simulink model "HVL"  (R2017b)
settings: Solver=FixedStepDiscrete  StartTime=0.0  StopTime=10.0  FixedStep=0.01  RelTol=1e-3  EnableMultiTasking=on
undefined symbols (not defined in the file): ASWTYPE_FALSE, ASWTYPE_TRUE, CcHVL_HvilSTGDutyThrd_pct, CcHVL_HvilSTVDutyThrd_pct, CcHVL_HVLSelfCheckTime_ms, CcHVL_PWMHighDuty_pct, CcHVL_PWMInHighPer_ms, CcHVL_PWMInLowPer_ms, CcHVL_PWMLowDuty_pct, CcHVL_PWMOutDuty_pct, CcHVL_PWMOutPer_us, Enum_MSMBMUState, HVL_CONST0_NUMB, HVL_CONST8_NUMB, HVL_CONST9_NUMB, HVL_RUNTIME_MS
libraries: AIWAYS_Powertrain_BMS_lib x11, simulink x1

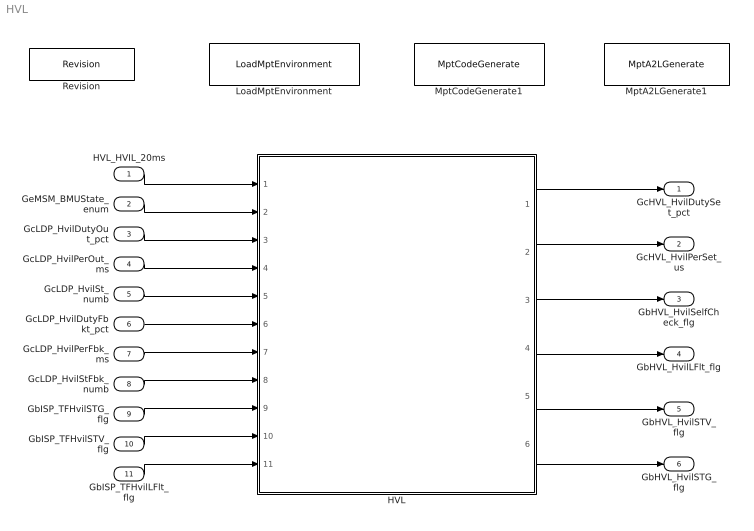
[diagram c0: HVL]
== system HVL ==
  HVL_HVIL_20ms : Inport
  GeMSM_BMUState_enum : Inport  Port=2
  GcLDP_HvilDutyOut_pct : Inport  Port=3
  GcLDP_HvilPerOut_ms : Inport  Port=4
  GcLDP_HvilSt_numb : Inport  Port=5
  GcLDP_HvilDutyFbkt_pct : Inport  Port=6
  GcLDP_HvilPerFbk_ms : Inport  Port=7
  GcLDP_HvilStFbk_numb : Inport  Port=8
  GbISP_TFHvilSTG_flg : Inport  Port=9
  GbISP_TFHvilSTV_flg : Inport  Port=10
  GbISP_TFHvilLFlt_flg : Inport  Port=11
  HVL : Subsystem
  LoadMptEnvironment : AIWAYS_Powertrain_BMS_lib/Config/LoadMptEnvironment  ProjectName=Comm  SuppierID=NewPlatformUAES
  MptA2LGenerate1 : AIWAYS_Powertrain_BMS_lib/Config/MptA2LGenerate  SystemSampleTime=-1
  MptCodeGenerate1 : AIWAYS_Powertrain_BMS_lib/Config/MptCodeGenerate  SystemSampleTime=-1
  Revision : AIWAYS_Powertrain_BMS_lib/Config/Revision  curVersion='M100C100'  newVersion='M100C100'
  GcHVL_HvilDutySet_pct : Outport
  GcHVL_HvilPerSet_us : Outport  Port=2
  GbHVL_HvilSelfCheck_flg : Outport  Port=3
  GbHVL_HvilLFlt_flg : Outport  Port=4
  GbHVL_HvilSTV_flg : Outport  Port=5
  GbHVL_HvilSTG_flg : Outport  Port=6
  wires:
  HVL_HVIL_20ms/1 -> HVL/1(HVL_HVIL_20ms)
  GeMSM_BMUState_enum/1 -> HVL/2(GeMSM_BMUState_enum)
  GcLDP_HvilDutyOut_pct/1 -> HVL/3(GcLDP_HvilDutyOut_pct)
  GcLDP_HvilPerOut_ms/1 -> HVL/4(GcLDP_HvilPerOut_ms)
  GcLDP_HvilSt_numb/1 -> HVL/5(GcLDP_HvilSt_numb)
  GcLDP_HvilDutyFbkt_pct/1 -> HVL/6(GcLDP_HvilDutyFbkt_pct)
  GcLDP_HvilPerFbk_ms/1 -> HVL/7(GcLDP_HvilPerFbk_ms)
  GcLDP_HvilStFbk_numb/1 -> HVL/8(GcLDP_HvilStFbk_numb)
  HVL/1(GcHVL_HvilDutySet_pct) -> GcHVL_HvilDutySet_pct/1
  HVL/2(GcHVL_HvilPerSet_us) -> GcHVL_HvilPerSet_us/1
  HVL/3(GbHVL_HvilSelfCheck_flg) -> GbHVL_HvilSelfCheck_flg/1
  HVL/4(GbHVL_HvilLFlt_flg) -> GbHVL_HvilLFlt_flg/1
  HVL/5(GbHVL_HvilSTV_flg) -> GbHVL_HvilSTV_flg/1
  HVL/6(GbHVL_HvilSTG_flg) -> GbHVL_HvilSTG_flg/1
  GbISP_TFHvilSTG_flg/1 -> HVL/9(GbISP_TFHvilSTG_flg)
  GbISP_TFHvilSTV_flg/1 -> HVL/10(GbISP_TFHvilSTV_flg)
  GbISP_TFHvilLFlt_flg/1 -> HVL/11(GbISP_TFHvilLFlt_flg)

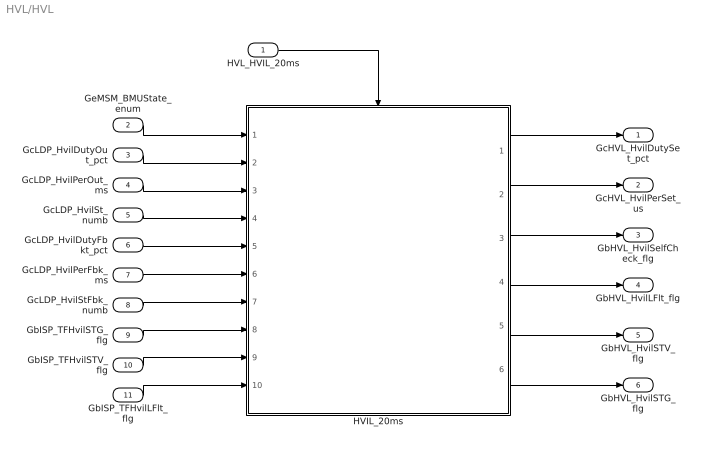
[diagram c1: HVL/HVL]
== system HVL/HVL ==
  HVL_HVIL_20ms : Inport
  GeMSM_BMUState_enum : Inport  Port=2
  GcLDP_HvilDutyOut_pct : Inport  Port=3
  GcLDP_HvilPerOut_ms : Inport  Port=4
  GcLDP_HvilSt_numb : Inport  Port=5
  GcLDP_HvilDutyFbkt_pct : Inport  Port=6
  GcLDP_HvilPerFbk_ms : Inport  Port=7
  GcLDP_HvilStFbk_numb : Inport  Port=8
  GbISP_TFHvilSTG_flg : Inport  Port=9
  GbISP_TFHvilSTV_flg : Inport  Port=10
  GbISP_TFHvilLFlt_flg : Inport  Port=11
  HVIL_20ms : Subsystem
  GcHVL_HvilDutySet_pct : Outport
  GcHVL_HvilPerSet_us : Outport  Port=2
  GbHVL_HvilSelfCheck_flg : Outport  Port=3
  GbHVL_HvilLFlt_flg : Outport  Port=4
  GbHVL_HvilSTV_flg : Outport  Port=5
  GbHVL_HvilSTG_flg : Outport  Port=6
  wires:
  HVL_HVIL_20ms/1 -> HVIL_20ms/Trigger
  GeMSM_BMUState_enum/1 -> HVIL_20ms/1(GeMSM_BMUState_enum)
  GcLDP_HvilDutyOut_pct/1 -> HVIL_20ms/2(GcLDP_HvilDutyOut_pct)
  GcLDP_HvilPerOut_ms/1 -> HVIL_20ms/3(GcLDP_HvilPerOut_ms)
  GcLDP_HvilSt_numb/1 -> HVIL_20ms/4(GcLDP_HvilSt_numb)
  GcLDP_HvilDutyFbkt_pct/1 -> HVIL_20ms/5(GcLDP_HvilDutyFbkt_pct)
  GcLDP_HvilPerFbk_ms/1 -> HVIL_20ms/6(GcLDP_HvilPerFbk_ms)
  GcLDP_HvilStFbk_numb/1 -> HVIL_20ms/7(GcLDP_HvilStFbk_numb)
  HVIL_20ms/3(GbHVL_HvilSelfCheck_flg) -> GbHVL_HvilSelfCheck_flg/1
  HVIL_20ms/2(GcHVL_HvilPerSet_us) -> GcHVL_HvilPerSet_us/1
  HVIL_20ms/4(GbHVL_HvilLFlt_flg) -> GbHVL_HvilLFlt_flg/1
  HVIL_20ms/1(GcHVL_HvilDutySet_pct) -> GcHVL_HvilDutySet_pct/1
  HVIL_20ms/5(GbHVL_HvilSTV_flg) -> GbHVL_HvilSTV_flg/1
  HVIL_20ms/6(GbHVL_HvilSTG_flg) -> GbHVL_HvilSTG_flg/1
  GbISP_TFHvilSTG_flg/1 -> HVIL_20ms/8(GbISP_TFHvilSTG_flg)
  GbISP_TFHvilSTV_flg/1 -> HVIL_20ms/9(GbISP_TFHvilSTV_flg)
  GbISP_TFHvilLFlt_flg/1 -> HVIL_20ms/10(GbISP_TFHvilLFlt_flg)

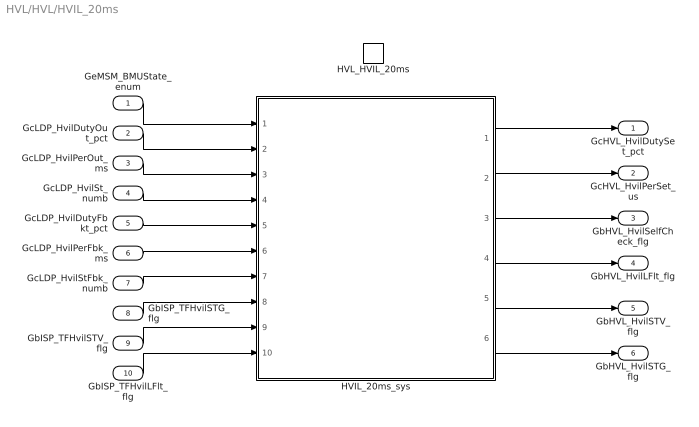
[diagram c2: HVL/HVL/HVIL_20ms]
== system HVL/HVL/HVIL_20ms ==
  GeMSM_BMUState_enum : Inport
  GcLDP_HvilDutyOut_pct : Inport  Port=2
  GcLDP_HvilPerOut_ms : Inport  Port=3
  GcLDP_HvilSt_numb : Inport  Port=4
  GcLDP_HvilDutyFbkt_pct : Inport  Port=5
  GcLDP_HvilPerFbk_ms : Inport  Port=6
  GcLDP_HvilStFbk_numb : Inport  Port=7
  GbISP_TFHvilSTG_flg : Inport  Port=8
  GbISP_TFHvilSTV_flg : Inport  Port=9
  GbISP_TFHvilLFlt_flg : Inport  Port=10
  HVL_HVIL_20ms : TriggerPort  TriggerType=function-call  VariantControl=(inherit)
  HVIL_20ms_sys : Subsystem
  GcHVL_HvilDutySet_pct : Outport
  GcHVL_HvilPerSet_us : Outport  Port=2
  GbHVL_HvilSelfCheck_flg : Outport  Port=3
  GbHVL_HvilLFlt_flg : Outport  Port=4
  GbHVL_HvilSTV_flg : Outport  Port=5
  GbHVL_HvilSTG_flg : Outport  Port=6
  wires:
  GeMSM_BMUState_enum/1 -> HVIL_20ms_sys/1(GeMSM_BMUState_enum)
  GcLDP_HvilDutyOut_pct/1 -> HVIL_20ms_sys/2(GcLDP_HvilDutyOut_pct)
  GcLDP_HvilPerOut_ms/1 -> HVIL_20ms_sys/3(GcLDP_HvilPerOut_ms)
  GcLDP_HvilSt_numb/1 -> HVIL_20ms_sys/4(GcLDP_HvilSt_numb)
  GcLDP_HvilDutyFbkt_pct/1 -> HVIL_20ms_sys/5(GcLDP_HvilDutyFbkt_pct)
  GcLDP_HvilPerFbk_ms/1 -> HVIL_20ms_sys/6(GcLDP_HvilPerFbk_ms)
  GcLDP_HvilStFbk_numb/1 -> HVIL_20ms_sys/7(GcLDP_HvilStFbk_numb)
  HVIL_20ms_sys/1(GcHVL_HvilDutySet_pct) -> GcHVL_HvilDutySet_pct/1
  HVIL_20ms_sys/2(GcHVL_HvilPerSet_us) -> GcHVL_HvilPerSet_us/1
  HVIL_20ms_sys/3(GbHVL_HvilSelfCheck_flg) -> GbHVL_HvilSelfCheck_flg/1
  HVIL_20ms_sys/4(GbHVL_HvilLFlt_flg) -> GbHVL_HvilLFlt_flg/1
  HVIL_20ms_sys/5(GbHVL_HvilSTV_flg) -> GbHVL_HvilSTV_flg/1
  HVIL_20ms_sys/6(GbHVL_HvilSTG_flg) -> GbHVL_HvilSTG_flg/1
  GbISP_TFHvilSTG_flg/1 -> HVIL_20ms_sys/8(GbISP_TFHvilSTG_flg)
  GbISP_TFHvilSTV_flg/1 -> HVIL_20ms_sys/9(GbISP_TFHvilSTV_flg)
  GbISP_TFHvilLFlt_flg/1 -> HVIL_20ms_sys/10(GbISP_TFHvilLFlt_flg)

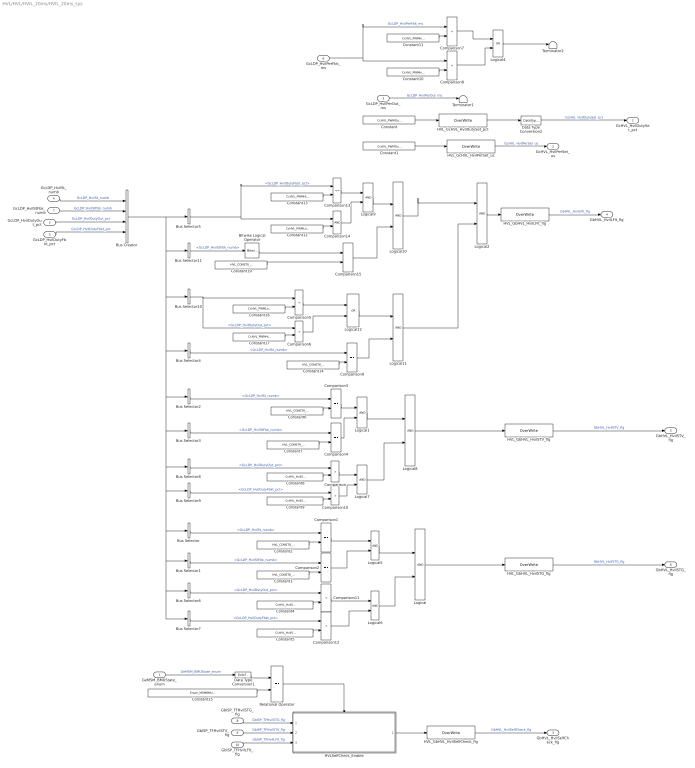
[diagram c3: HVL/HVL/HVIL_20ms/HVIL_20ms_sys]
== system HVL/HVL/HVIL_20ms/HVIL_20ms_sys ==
  GeMSM_BMUState_enum : Inport
  GcLDP_HvilDutyOut_pct : Inport  Port=2
  GcLDP_HvilPerOut_ms : Inport  Port=3
  GcLDP_HvilSt_numb : Inport  Port=4
  GcLDP_HvilDutyFbkt_pct : Inport  Port=5
  GcLDP_HvilPerFbk_ms : Inport  Port=6
  GcLDP_HvilStFbk_numb : Inport  Port=7
  GbISP_TFHvilSTG_flg : Inport  Port=8
  GbISP_TFHvilSTV_flg : Inport  Port=9
  GbISP_TFHvilLFlt_flg : Inport  Port=10
  Bitwise Logical Operator : simulink/Logic and Bit Operations/Bitwise Operator  logicop=AND  UseBitMask=on  BitMask=HVL_CONST24_NUMB  BitMaskRealWorld=Stored Integer
  Bus Creator : BusCreator  Inputs=4
  Bus Selector : BusSelector  OutputSignals=GcLDP_HvilSt_numb
  Bus Selector1 : BusSelector  OutputSignals=GcLDP_HvilStFbk_numb
  Bus Selector10 : BusSelector  OutputSignals=GcLDP_HvilDutyOut_pct
  Bus Selector11 : BusSelector  OutputSignals=GcLDP_HvilStFbk_numb
  Bus Selector2 : BusSelector  OutputSignals=GcLDP_HvilSt_numb
  Bus Selector3 : BusSelector  OutputSignals=GcLDP_HvilStFbk_numb
  Bus Selector4 : BusSelector  OutputSignals=GcLDP_HvilSt_numb
  Bus Selector5 : BusSelector  OutputSignals=GcLDP_HvilDutyFbkt_pct
  Bus Selector6 : BusSelector  OutputSignals=GcLDP_HvilDutyOut_pct
  Bus Selector7 : BusSelector  OutputSignals=GcLDP_HvilDutyFbkt_pct
  Bus Selector8 : BusSelector  OutputSignals=GcLDP_HvilDutyOut_pct
  Bus Selector9 : BusSelector  OutputSignals=GcLDP_HvilDutyFbkt_pct
  Comparison{,6,8,10} (4 alike) : RelationalOperator  Operator=>  OutDataTypeStr=boolean
  Comparison{1..4,9,15} (6 alike) : RelationalOperator  Operator===  OutDataTypeStr=boolean
  Comparison{5,7,11..12} (4 alike) : RelationalOperator  Operator=<  OutDataTypeStr=boolean
  Comparison13 : RelationalOperator  Operator=<=  OutDataTypeStr=boolean
  Comparison14 : RelationalOperator  OutDataTypeStr=boolean
  Constant : Constant  Value=CcHVL_PWMOutDuty_pct
  Constant1 : Constant  Value=CcHVL_PWMOutPer_us
  Constant10 : Constant  Value=CcHVL_PWMInHighPer_ms
  Constant11 : Constant  Value=CcHVL_PWMInLowPer_ms
  Constant12 : Constant  Value=CcHVL_PWMLowDuty_pct
  Constant13 : Constant  Value=CcHVL_PWMHighDuty_pct
  Constant14 : Constant  Value=HVL_CONST8_NUMB
  Constant15 : Constant  Value=Enum_MSMBMUState.Enum_MSMBMUState_Standby
  Constant16 : Constant  Value=CcHVL_PWMLowDuty_pct
  Constant17 : Constant  Value=CcHVL_PWMHighDuty_pct
  Constant19 : Constant  Value=HVL_CONST0_NUMB
  Constant2 : Constant  Value=HVL_CONST8_NUMB
  Constant3 : Constant  Value=HVL_CONST8_NUMB
  Constant4 : Constant  Value=CcHVL_HvilSTGDutyThrd_pct
  Constant5 : Constant  Value=CcHVL_HvilSTGDutyThrd_pct
  Constant6 : Constant  Value=HVL_CONST9_NUMB
  Constant7 : Constant  Value=HVL_CONST9_NUMB
  Constant8 : Constant  Value=CcHVL_HvilSTVDutyThrd_pct
  Constant9 : Constant  Value=CcHVL_HvilSTVDutyThrd_pct
  Data Type Conversion1 : DataTypeConversion
  Data Type Conversion2 : DataTypeConversion
  HVLSelfCheck_Enable : Subsystem
  HVL_GbHVL_HvilLFlt_flg : AIWAYS_Powertrain_BMS_lib/Signals/OverWrite  OverWrite_Value=CbHVL_HvilLFltOvr_flg  OverWrite_flag=CbHVL_HvilLFltOvrSwt_flg
  HVL_GbHVL_HvilSTG_flg : AIWAYS_Powertrain_BMS_lib/Signals/OverWrite  OverWrite_Value=CbHVL_HvilSTGOvr_flg  OverWrite_flag=CbHVL_HvilSTGOvrSwt_flg
  HVL_GbHVL_HvilSTV_flg : AIWAYS_Powertrain_BMS_lib/Signals/OverWrite  OverWrite_Value=CbHVL_HvilSTVOvr_flg  OverWrite_flag=CbHVL_HvilSTVOvrSwt_flg
  HVL_GbHVL_HvilSelfCheck_flg : AIWAYS_Powertrain_BMS_lib/Signals/OverWrite  OverWrite_Value=CbHVL_HvilSelfCheckOvr_flg  OverWrite_flag=CbHVL_HvilSelfCheckOvrSwt_flg
  HVL_GcHVL_HvilDutySet_pct : AIWAYS_Powertrain_BMS_lib/Signals/OverWrite  OverWrite_Value=CcHVL_HvilDutySetOvr_pct  OverWrite_flag=CbHVL_HvilDutySetOvrSwt_flg
  HVL_GcHVL_HvilPerSet_us : AIWAYS_Powertrain_BMS_lib/Signals/OverWrite  OverWrite_Value=CcHVL_HvilPerSetOvr_us  OverWrite_flag=CbHVL_HvilPerSetOvrSwt_flg
  Logical{,1..2,5..11} (10 alike) : Logic  OutDataTypeStr=boolean
  Logical12 : Logic  Operator=OR  OutDataTypeStr=boolean
  Logical4 : Logic  Operator=OR  OutDataTypeStr=boolean
  Relational Operator : RelationalOperator  Operator===  OutDataTypeStr=boolean
  Terminator1 : Terminator
  Terminator2 : Terminator
  GcHVL_HvilDutySet_pct : Outport
  GcHVL_HvilPerSet_us : Outport  Port=2
  GbHVL_HvilSelfCheck_flg : Outport  Port=3
  GbHVL_HvilLFlt_flg : Outport  Port=4
  GbHVL_HvilSTV_flg : Outport  Port=5
  GbHVL_HvilSTG_flg : Outport  Port=6
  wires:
  GeMSM_BMUState_enum/1 -> Data Type Conversion1/1  "GeMSM_BMUState_enum"
  GcLDP_HvilPerOut_ms/1 -> Terminator1/1  "GcLDP_HvilPerOut_ms"
  GcLDP_HvilSt_numb/1 -> Bus Creator/1  "GcLDP_HvilSt_numb"
  GcLDP_HvilDutyFbkt_pct/1 -> Bus Creator/4  "GcLDP_HvilDutyFbkt_pct"
  GcLDP_HvilPerFbk_ms/1 -> Comparison7/1, Comparison8/1  "GcLDP_HvilPerFbk_ms"
  GcLDP_HvilStFbk_numb/1 -> Bus Creator/2  "GcLDP_HvilStFbk_numb"
  Data Type Conversion2/1 -> GcHVL_HvilDutySet_pct/1  "GcHVL_HvilDutySet_pct"
  HVL_GcHVL_HvilPerSet_us/1 -> GcHVL_HvilPerSet_us/1  "GcHVL_HvilPerSet_us"
  HVL_GbHVL_HvilSelfCheck_flg/1 -> GbHVL_HvilSelfCheck_flg/1  "GbHVL_HvilSelfCheck_flg"
  HVL_GbHVL_HvilLFlt_flg/1 -> GbHVL_HvilLFlt_flg/1  "GbHVL_HvilLFlt_flg"
  HVL_GbHVL_HvilSTV_flg/1 -> GbHVL_HvilSTV_flg/1  "GbHVL_HvilSTV_flg"
  HVL_GbHVL_HvilSTG_flg/1 -> GbHVL_HvilSTG_flg/1  "GbHVL_HvilSTG_flg"
  Constant1/1 -> HVL_GcHVL_HvilPerSet_us/1
  HVLSelfCheck_Enable/1(GbHVL_HvilSelfCheck_flg) -> HVL_GbHVL_HvilSelfCheck_flg/1
  Logical2/1 -> HVL_GbHVL_HvilLFlt_flg/1
  Logical8/1 -> HVL_GbHVL_HvilSTV_flg/1
  Logical/1 -> HVL_GbHVL_HvilSTG_flg/1
  Constant2/1 -> Comparison1/2
  Constant3/1 -> Comparison2/2
  Comparison1/1 -> Logical5/1
  Comparison2/1 -> Logical5/2
  Bus Selector/1 -> Comparison1/1  "<GcLDP_HvilSt_numb>"
  Bus Selector1/1 -> Comparison2/1  "<GcLDP_HvilStFbk_numb>"
  Bus Selector3/1 -> Comparison4/1  "<GcLDP_HvilStFbk_numb>"
  Bus Selector2/1 -> Comparison3/1  "<GcLDP_HvilSt_numb>"
  Bus Creator/1 -> Bus Selector5/1, Bus Selector8/1, Bus Selector7/1, Bus Selector6/1, Bus Selector1/1, Bus Selector/1, Bus Selector9/1, Bus Selector3/1, Bus Selector2/1, Bus Selector4/1, Bus Selector10/1, Bus Selector11/1
  Comparison4/1 -> Logical1/2
  Comparison3/1 -> Logical1/1
  Constant7/1 -> Comparison4/2
  Constant6/1 -> Comparison3/2
  GcLDP_HvilDutyOut_pct/1 -> Bus Creator/3  "GcLDP_HvilDutyOut_pct"
  Constant10/1 -> Comparison8/2
  Constant11/1 -> Comparison7/2
  Constant12/1 -> Comparison14/2
  Constant13/1 -> Comparison13/2
  Constant14/1 -> Comparison9/2
  Bus Selector4/1 -> Comparison9/1  "<GcLDP_HvilSt_numb>"
  Comparison9/1 -> Logical11/2
  Data Type Conversion1/1 -> Relational Operator/1
  Constant15/1 -> Relational Operator/2
  Relational Operator/1 -> HVLSelfCheck_Enable/Enable
  Comparison13/1 -> Logical9/1
  Comparison14/1 -> Logical9/2
  Logical9/1 -> Logical10/1
  Comparison7/1 -> Logical4/1
  Comparison8/1 -> Logical4/2
  Logical4/1 -> Terminator2/1
  Bus Selector5/1 -> Comparison13/1, Comparison14/1  "<GcLDP_HvilDutyFbkt_pct>"
  Constant4/1 -> Comparison11/2
  Bus Selector6/1 -> Comparison11/1  "<GcLDP_HvilDutyOut_pct>"
  Bus Selector7/1 -> Comparison12/1  "<GcLDP_HvilDutyFbkt_pct>"
  Constant5/1 -> Comparison12/2
  Comparison11/1 -> Logical6/1
  Comparison12/1 -> Logical6/2
  Logical5/1 -> Logical/1
  Logical6/1 -> Logical/2
  Bus Selector8/1 -> Comparison/1  "<GcLDP_HvilDutyOut_pct>"
  Constant8/1 -> Comparison/2
  Constant9/1 -> Comparison10/2
  Bus Selector9/1 -> Comparison10/1  "<GcLDP_HvilDutyFbkt_pct>"
  Comparison/1 -> Logical7/1
  Comparison10/1 -> Logical7/2
  Logical1/1 -> Logical8/1
  Logical7/1 -> Logical8/2
  Bus Selector10/1 -> Comparison6/1, Comparison5/1  "<GcLDP_HvilDutyOut_pct>"
  Constant16/1 -> Comparison5/2
  Constant17/1 -> Comparison6/2
  Comparison5/1 -> Logical12/1
  Comparison6/1 -> Logical12/2
  Logical12/1 -> Logical11/1
  Constant19/1 -> Comparison15/2
  Bus Selector11/1 -> Bitwise Logical Operator/1  "<GcLDP_HvilStFbk_numb>"
  Bitwise Logical Operator/1 -> Comparison15/1
  Comparison15/1 -> Logical10/2
  Logical10/1 -> Logical2/1
  Logical11/1 -> Logical2/2
  GbISP_TFHvilLFlt_flg/1 -> HVLSelfCheck_Enable/3(GbISP_TFHvilLFlt_flg)  "GbISP_TFHvilLFlt_flg"
  GbISP_TFHvilSTG_flg/1 -> HVLSelfCheck_Enable/1(GbISP_TFHvilSTG_flg)  "GbISP_TFHvilSTG_flg"
  GbISP_TFHvilSTV_flg/1 -> HVLSelfCheck_Enable/2(GbISP_TFHvilSTV_flg)  "GbISP_TFHvilSTV_flg"
  Constant/1 -> HVL_GcHVL_HvilDutySet_pct/1
  HVL_GcHVL_HvilDutySet_pct/1 -> Data Type Conversion2/1

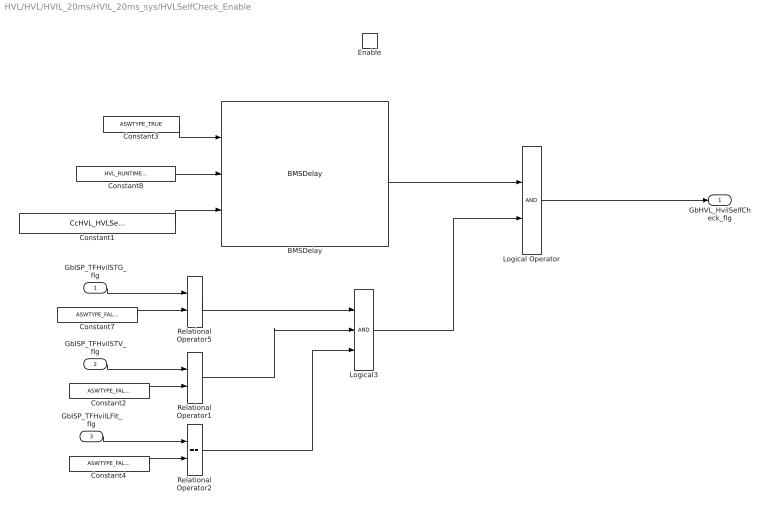
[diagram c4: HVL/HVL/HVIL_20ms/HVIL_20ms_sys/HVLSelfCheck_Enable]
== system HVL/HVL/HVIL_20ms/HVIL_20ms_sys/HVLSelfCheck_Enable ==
  GbISP_TFHvilSTG_flg : Inport
  GbISP_TFHvilSTV_flg : Inport  Port=2
  GbISP_TFHvilLFlt_flg : Inport  Port=3
  Enable : EnablePort  StatesWhenEnabling=reset
  BMSDelay : AIWAYS_Powertrain_BMS_lib/Debounce & Delay/BMSDelay
  Constant1 : Constant  Value=CcHVL_HVLSelfCheckTime_ms
  Constant2 : Constant  Value=ASWTYPE_FALSE
  Constant3 : Constant  Value=ASWTYPE_TRUE
  Constant4 : Constant  Value=ASWTYPE_FALSE
  Constant7 : Constant  Value=ASWTYPE_FALSE
  Constant8 : Constant  Value=HVL_RUNTIME_MS
  Logical Operator : Logic  AllPortsSameDT=off  OutDataTypeStr=boolean
  Logical3 : Logic  Inputs=3  OutDataTypeStr=boolean
  Relational Operator1 : RelationalOperator  Operator===  OutDataTypeStr=boolean
  Relational Operator2 : RelationalOperator  Operator===  OutDataTypeStr=boolean
  Relational Operator5 : RelationalOperator  Operator===  OutDataTypeStr=boolean
  GbHVL_HvilSelfCheck_flg : Outport
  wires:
  Constant8/1 -> BMSDelay/2
  Constant1/1 -> BMSDelay/3
  BMSDelay/1 -> Logical Operator/1
  Constant3/1 -> BMSDelay/1
  Constant7/1 -> Relational Operator5/2
  Logical Operator/1 -> GbHVL_HvilSelfCheck_flg/1
  GbISP_TFHvilSTG_flg/1 -> Relational Operator5/1
  GbISP_TFHvilSTV_flg/1 -> Relational Operator1/1
  Constant2/1 -> Relational Operator1/2
  Constant4/1 -> Relational Operator2/2
  GbISP_TFHvilLFlt_flg/1 -> Relational Operator2/1
  Relational Operator5/1 -> Logical3/1
  Relational Operator1/1 -> Logical3/2
  Relational Operator2/1 -> Logical3/3
  Logical3/1 -> Logical Operator/2
